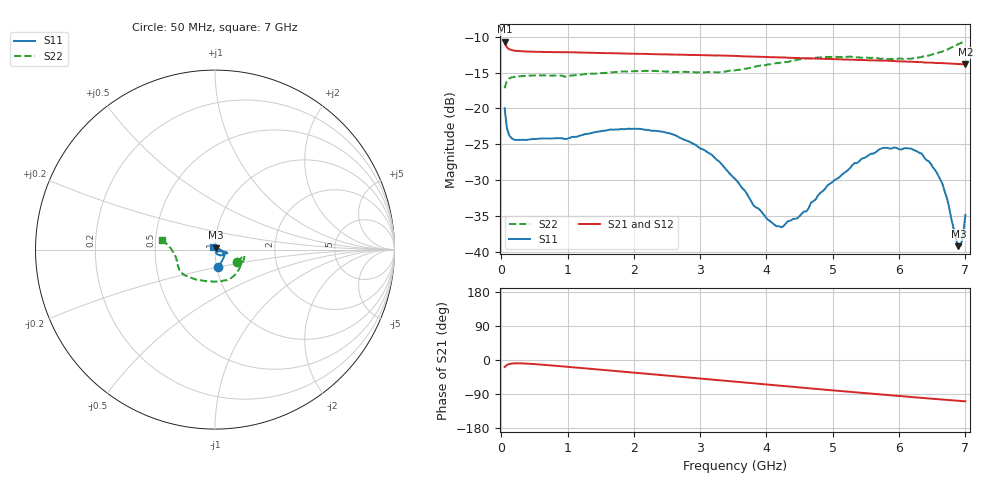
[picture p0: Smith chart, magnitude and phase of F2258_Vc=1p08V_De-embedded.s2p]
! Integrated Device Technology
! Corporate Headquarters
! 6024 Silver Creek Valley Road
! San Jose, CA 95138  USA
! Phone:  1-408-284-8200
! Toll Free:  1-800-223-1366
! Webpage:  http://www.idt.com/
! Timing and RF Division
! 515 Groton Road, Suite 102
! Westford, MA 01886-6024
! Device:  F2258
! Description: Voltage Variable RF Attenuator
! Frequency:  50.0 -  6000.00 MHz
! Package:  3x3 mm Thin QFN Plastic Package: 16 pin
! Ports:  2 RF, 2 DC
!  Pin  1  = NC
!  Pin  2  = NC
!  Pin  3  = RF2  = Port 2
!  Pin  4  = GND
!  Pin  5  = Vdd
!  Pin  6  = NC
!  Pin  7  = VCTRL
!  Pin  8  = NC
!  Pin  9  = GND
!  Pin 10  = RF1  = Port 1
!  Pin 11  = NC
!  Pin 12  = NC
!  Pin 13  = NC
!  Pin 14  = NC
!  Pin 15  = NC
!  Pin 16  = NC
! Vcntrl:  1.080 Volts
! Vdd:  +3.300 Volts
! Current:  1.161 mA
! Data:  The device was measured on a the F2258 evaluation board which has
!  individual transmission lines to the RF pins.  Data was collected
!  using a calibrated network analyzer.  The evaluation board was
!  de-embedded using a TRL calibration technique.
!  The reference plane is the edge of the package pin.
! Misc:  SN 10
!  Action Tracker AT0285
! Date Measured:  2014-12-10
! Date:  2016-01-13  MJV
! Note:
!  Integrated Device Technology supplies this data as a sample of measured
!  data at the package pin for this product.  Your particular data for this
!  product may vary.
!  Data was taken at 25 degrees C.
!  Integrated Device Technology reserves the right to change this data at anytime.
!Freq_(GHz)  S11M_(dB)  S11P_(deg)  S21M_(dB)  S21P_(deg)  S12M_(dB)  S12P_(deg)  S22M_(dB)  S22P_(deg)
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# GHz S dB R 50
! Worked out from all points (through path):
!   201 points, 50 MHz to 7 GHz, reference 50 ohm
!   highest |S21| = -10.69 dB at 50 MHz (marker M1); lowest = -13.9 dB at 7 GHz (marker M2)
!   group delay of S21, straight-line fit = 42.1 ps
!   lowest |S11| = -39.2 dB at 6.896 GHz (marker M3), VSWR 1.02, Z = 50.4 + j1.04 ohm
!   |S11| at or under -10 dB: start of sweep to end of sweep
!   |S22| runs from -17.2 to -10.5 dB; largest |S21 - S12| = 0.0012
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0.05  -19.96 -80.1  -10.69 -18.5  -10.69 -18.5  -17.20 -29.1
0.08475  -22.79 -55.6  -11.49 -13.1  -11.47 -13.1  -16.16 -16.2
0.189  -24.36 -26.9  -11.93 -8.9  -11.91 -8.9  -15.61 -11.6
1.2315  -23.70 -17.9  -12.22 -21.5  -12.24 -21.5  -15.25 -38.7
1.9265  -22.84 -15.9  -12.36 -32.2  -12.38 -32.1  -14.83 -56.6
2.37825  -23.21 -14.2  -12.45 -39.1  -12.45 -39.1  -14.79 -68.5
3.07325  -25.89 -13.0  -12.58 -50.1  -12.58 -50.1  -14.98 -91.3
3.525  -29.84 -16.9  -12.70 -57.3  -12.70 -57.3  -14.69 -109.2
3.803  -33.55 -28.3  -12.78 -61.8  -12.77 -61.8  -14.22 -119.9
4.1505  -36.45 -50.2  -12.87 -67.2  -12.88 -67.2  -13.69 -130.3
4.46325  -35.38 -70.3  -12.98 -72.1  -12.98 -72.1  -13.23 -138.5
4.7065  -32.95 -67.5  -13.04 -75.7  -13.04 -75.7  -13.00 -142.8
5.332  -27.63 -48.4  -13.22 -85.1  -13.21 -85.1  -12.90 -152.1
5.85325  -25.61 -32.9  -13.38 -92.8  -13.37 -92.8  -13.10 -161.9
6.20075  -25.71 -23.9  -13.50 -97.9  -13.50 -97.9  -13.04 -170.4
6.47875  -27.75 -12.5  -13.61 -101.9  -13.63 -101.9  -12.54 -177.5
6.6525  -30.52 -0.7  -13.69 -104.4  -13.71 -104.3  -12.06 177.5
6.722  -32.53 7.2  -13.73 -105.4  -13.73 -105.4  -11.83 175.5
6.89575  -39.24 70.7  -13.82 -107.7  -13.83 -107.7  -11.01 171.8
6.9305  -39.17 91.2  -13.82 -108.1  -13.84 -108.1  -10.89 171.4
6.96525  -37.66 111.9  -13.86 -108.7  -13.85 -108.6  -10.73 170.4
7  -34.88 123.3  -13.86 -109.1  -13.85 -109.1  -10.52 169.6
